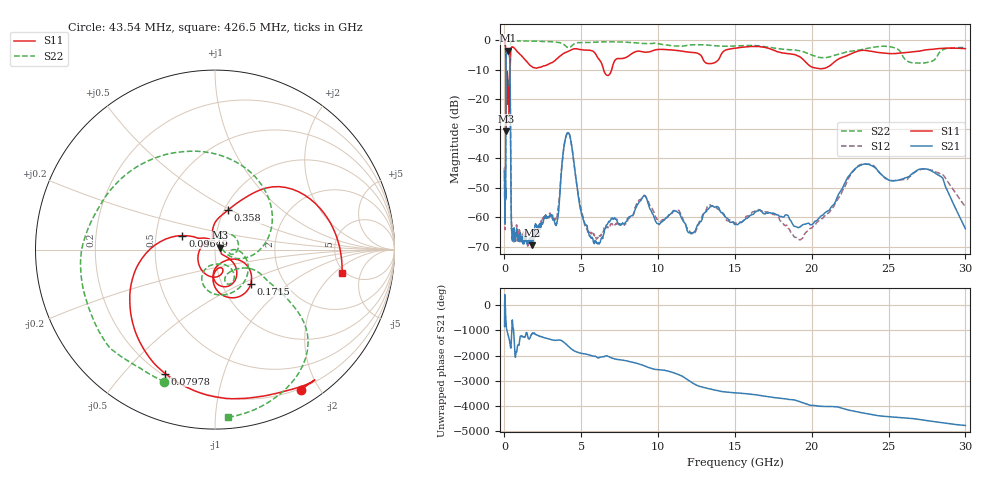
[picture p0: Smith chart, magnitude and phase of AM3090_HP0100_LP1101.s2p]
! Date/Time: Thu, Feb 28, 2019 1:58 PM
! Network Analyzer: Agilent Technologies E8364B Rev: A.07.50.67
! Sweep from 0.010 to 30.000 GHz, 1601 Points, Sweep Type: LOG
! Power Supply: 5.023 V, 0.002 A
# Hz S DB R 50
!freq MagS11 AngS11 MagS21 AngS21 MagS12 AngS12 MagS22 AngS22
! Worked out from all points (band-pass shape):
!   1601 points, 10 MHz to 30 GHz, reference 50 ohm
!   highest |S21| = -3.58 dB at 236.3 MHz (marker M1); lowest = -69.6 dB at 1.82 GHz (marker M2)
!   |S21| within 3 dB of the highest: 107 MHz to 343.9 MHz (236.9 MHz wide, 105 % of centre)
!   lowest |S11| = -30.9 dB at 103.5 MHz (marker M3), VSWR 1.06, Z = 52.7 + j1.07 ohm
!   |S11| at or under -10 dB: 94.44 MHz to 369.9 MHz (275.5 MHz wide, 119 % of centre); 6.455 GHz to 6.978 GHz (522.7 MHz wide, 7.78 % of centre)
!   |S22| runs from -30.2 to -0.1 dB; largest |S21 - S12| = 0.012
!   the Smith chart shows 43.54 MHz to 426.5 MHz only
!   S11 on the Smith chart (normalised r, x): 43.54 MHz: 0.18, -1.77; 79.78 MHz: 0.21, -0.65; 96.49 MHz: 0.69, +0.11; 171.5 MHz: 1.37, -0.56; 358 MHz: 1.04, +0.48; 426.5 MHz: 4.67, -2.58
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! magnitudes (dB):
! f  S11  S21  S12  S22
! 10 MHz  -0.2  -46.5  -43.4  -0.7
! 38.04 MHz  -0.5  -60.7  -59.4  -1.7
! 43.54 MHz  -0.8  -60.8  -62.6  -2.1
! 79.78 MHz  -2.6  -47.2  -47.3  -4.6
! 96.49 MHz  -14.1  -14.1  -14.1  -14.1
! 103.5 MHz  -30.9  -7.8  -7.8  -29.6
! 119.1 MHz  -13.5  -5.0  -5.0  -18.2
! 144.7 MHz  -21.5  -3.8  -3.8  -21.8
! 171.5 MHz  -11.2  -3.7  -3.6  -13.4
! 236.3 MHz  -19.6  -3.6  -3.6  -18.2
! 358 MHz  -12.7  -8.8  -8.7  -8.5
! 426.5 MHz  -2.8  -53.2  -52.6  -0.6
! 550.5 MHz  -2.4  -65.0  -64.8  -0.2
! 1.82 GHz  -9.1  -69.6  -67.0  -0.3
! 2.084 GHz  -9.5  -62.8  -64.7  -0.4
! 3.385 GHz  -6.4  -62.1  -60.5  -0.7
! 4.115 GHz  -3.9  -31.4  -31.3  -2.5
! 5.64 GHz  -3.5  -67.2  -65.5  -0.8
! 7.926 GHz  -5.8  -61.5  -62.2  -0.7
! 19.41 GHz  -6.4  -62.6  -67.1  -3.8
! 23.48 GHz  -3.5  -41.9  -42.1  -3.0
! 30 GHz  -2.9  -64.0  -56.5  -2.5
